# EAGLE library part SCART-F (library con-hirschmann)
TV SCART CONNECTOR
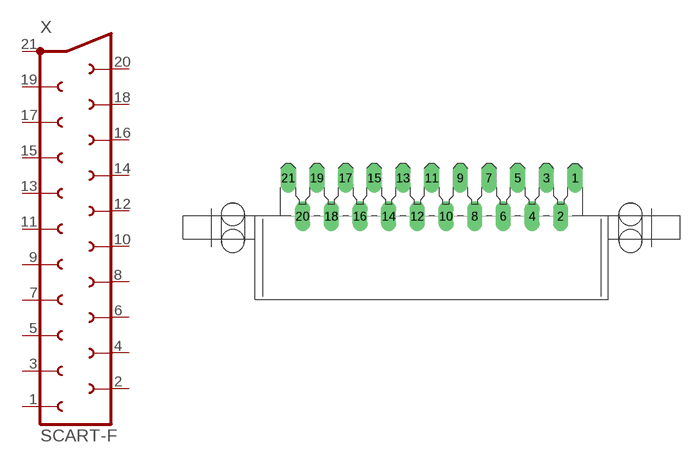
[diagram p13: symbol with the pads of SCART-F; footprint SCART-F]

Designator prefix X

## SCART-F (OC_FARNELL: unknown; OC_NEWARK: unknown)  [SCART-F]
1  1  pas
2  2  pas
3  3  pas
4  4  pas
5  5  pas
6  6  pas
7  7  pas
8  8  pas
9  9  pas
10  10  pas
11  11  pas
12  12  pas
13  13  pas
14  14  pas
15  15  pas
16  16  pas
17  17  pas
18  18  pas
19  19  pas
20  20  pas
21  21  pas

## Footprint SCART-F (pad centres in mm)
TV SCART CONNECTOR
drill 1.321 long: 1 19.05,5.08; 2 17.145,0; 3 15.24,5.08; 4 13.335,0; 5 11.43,5.08; 6 9.525,0; 7 7.62,5.08; 8 5.715,0; 9 3.81,5.08; 10 1.905,0; 11 0,5.08; 12 -1.905,0; 13 -3.81,5.08; 14 -5.715,0; 15 -7.62,5.08; 16 -9.525,0; 17 -11.43,5.08; 18 -13.335,0; 19 -15.24,5.08; 20 -17.145,0; 21 -19.05,5.08
hole 3.023 at 26.416,0.254
hole 3.023 at 26.416,-3.302
hole 3.023 at -26.416,0.254
hole 3.023 at -26.416,-3.302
